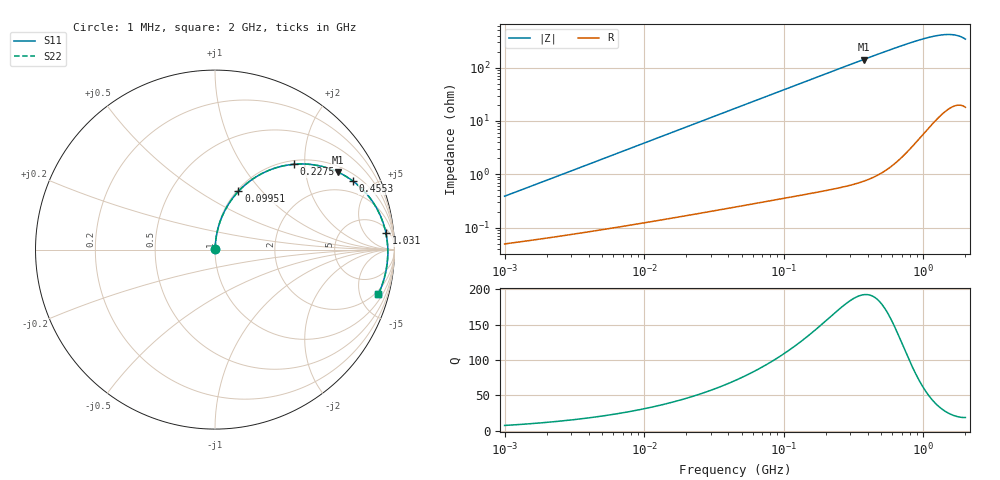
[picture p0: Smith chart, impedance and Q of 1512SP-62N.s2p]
!AWR Design Environment (3650) Tue Sep 29 15:25:04 2020
!freq-unit  param-type  data-format  keyword  impedance-ohms
# MHz  S  MA  R  50
!Freq  MagS11  AngS11  MagS21  AngS21  MagS12  AngS12  MagS22  AngS22
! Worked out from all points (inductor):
!   801 points, 1 MHz to 2 GHz, reference 50 ohm
!   read as one part in series: L = 61.3 nH near 1.039 MHz
!   highest Q = 192 at 372.9 MHz (marker M1), where L = 60.6 nH
!   S11 on the Smith chart (normalised r, x): 1 MHz: 1.00, +0.01; 99.51 MHz: 1.02, +0.75; 227.5 MHz: 1.08, +1.76; 455.3 MHz: 1.32, +3.84; 1.031 GHz: 8, +17; 2 GHz: 1.57, -7.09
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1  0.003803 82.3  0.9995 -0.2  0.9995 -0.2  0.003803 82.3
3.573795  0.01349 85.8  0.9991 -0.8  0.9991 -0.8  0.01349 85.8
7.152559  0.02697 86.1  0.9986 -1.6  0.9986 -1.6  0.02696 86.1
12.65119  0.04763 85.5  0.9975 -2.8  0.9975 -2.8  0.04762 85.5
25.08046  0.09404 83.3  0.9937 -5.6  0.9937 -5.6  0.09403 83.3
44.78507  0.1662 79.2  0.9837 -10.0  0.9837 -10.0  0.1662 79.2
69.34475  0.2523 74.1  0.9648 -15.2  0.9648 -15.2  0.2523 74.1
99.51103  0.3502 68.1  0.9334 -21.4  0.9334 -21.4  0.3501 68.1
126.2022  0.4282 63.0  0.9002 -26.5  0.9002 -26.5  0.428 63.0
160.0527  0.5146 57.2  0.8537 -32.4  0.8537 -32.4  0.5144 57.2
191.7307  0.5833 52.2  0.8084 -37.4  0.8084 -37.4  0.5831 52.2
227.5059  0.648 47.2  0.7577 -42.4  0.7577 -42.4  0.6478 47.2
291.2838  0.7356 39.7  0.6734 -50.0  0.6734 -50.0  0.7353 39.7
372.9409  0.8104 32.2  0.5819 -57.5  0.5819 -57.5  0.81 32.2
455.3282  0.8589 26.3  0.5079 -63.4  0.5079 -63.4  0.8584 26.3
566.5845  0.8996 20.3  0.4317 -69.3  0.4317 -69.3  0.899 20.3
760.7247  0.9363 12.8  0.3431 -76.7  0.3431 -76.7  0.9356 12.8
1031.141  0.957 5.5  0.2741 -83.5  0.2741 -83.5  0.9562 5.5
1283.094  0.963 0.1  0.2424 -88.2  0.2424 -88.2  0.9623 0.1
1522.507  0.9625 -4.6  0.2327 -92.2  0.2327 -92.2  0.9619 -4.6
1739.198  0.9575 -9.0  0.2403 -96.1  0.2403 -96.1  0.957 -9.0
2000  0.9432 -15.3  0.276 -102.1  0.276 -102.1  0.9431 -15.4
